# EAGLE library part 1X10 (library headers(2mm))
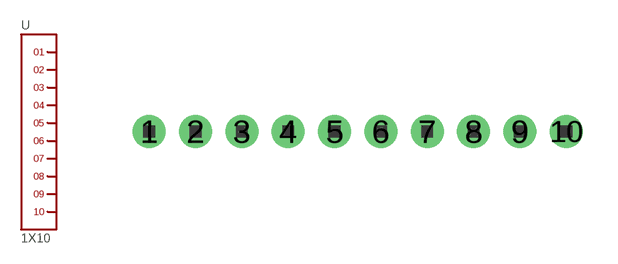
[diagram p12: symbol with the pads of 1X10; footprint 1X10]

Designator prefix -

## 1X10  [1X10]
1  1
2  2
3  3
4  4
5  5
6  6
7  7
8  8
9  9
10  10

## Footprint 1X10 (pad centres in mm)
drill 0.8 pad 1.422: 1 -9,0; 2 -7,0; 3 -5,0; 4 -3,0; 5 -1,0; 6 1,0; 7 3,0; 8 5,0; 9 7,0; 10 9,0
